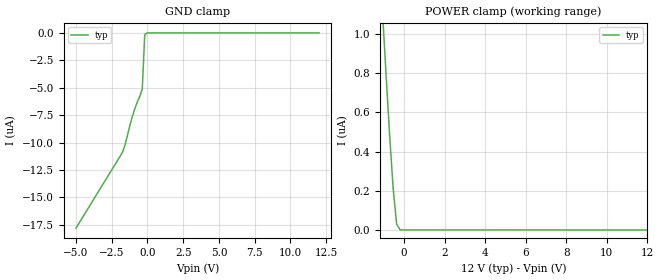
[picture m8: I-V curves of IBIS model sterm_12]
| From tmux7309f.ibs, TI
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| sterm_12
[Model]   sterm_12
Model_type   Terminator
|   typ   min   max
C_comp   1.598234e-12   NA   NA
[Voltage Range]   12   NA   NA
[Temperature Range]   27   NA   NA
[Power Clamp Reference]   12   NA   NA
[GND Clamp Reference]   0   NA   NA
[GND Clamp]
|   Voltage   I(typ)   I(min)   I(max)
-5V       -17.8uA    NA         NA
-1.737V   -10.85uA   NA         NA
-1.566V   -10.2uA    NA         NA
-1.222V   -8.405uA   NA         NA
-1.051V   -7.596uA   NA         NA
-878.8mV  -6.891uA   NA         NA
-535.4mV  -5.783uA   NA         NA
-363.6mV  -5.105uA   NA         NA
-191.9mV  -142nA     NA         NA
-20.2mV   -285.8pA   NA         NA
12V       268.1pA    NA         NA
[POWER Clamp]
|   Voltage   I(typ)   I(min)   I(max)
-5V       8.864uA    NA         NA
-1.05V    1.093uA    NA         NA
-878.8mV  780.4nA    NA         NA
-707.1mV  480.8nA    NA         NA
-535.4mV  210.2nA    NA         NA
-363.6mV  29.21nA    NA         NA
-191.9mV  617.3pA    NA         NA
12V       -178.9pA   NA         NA
